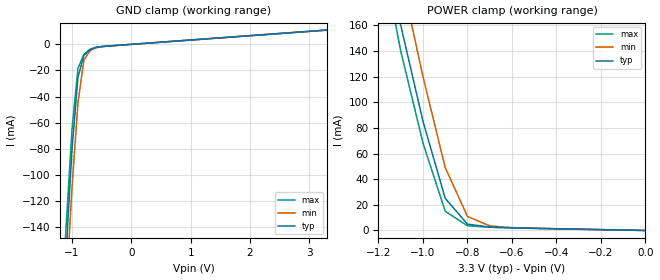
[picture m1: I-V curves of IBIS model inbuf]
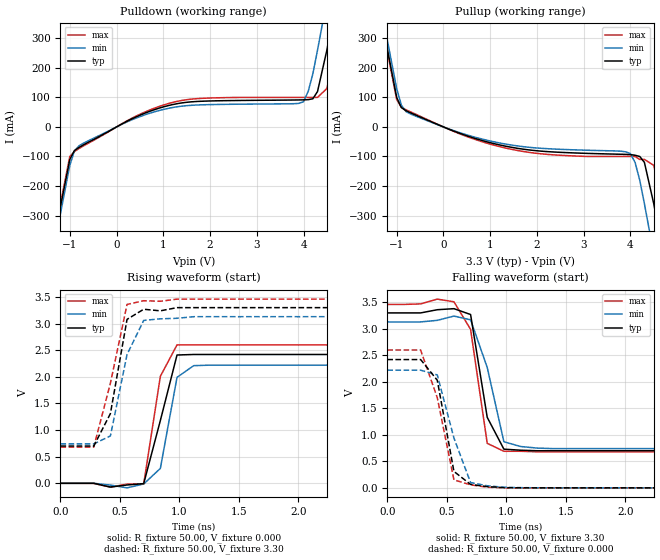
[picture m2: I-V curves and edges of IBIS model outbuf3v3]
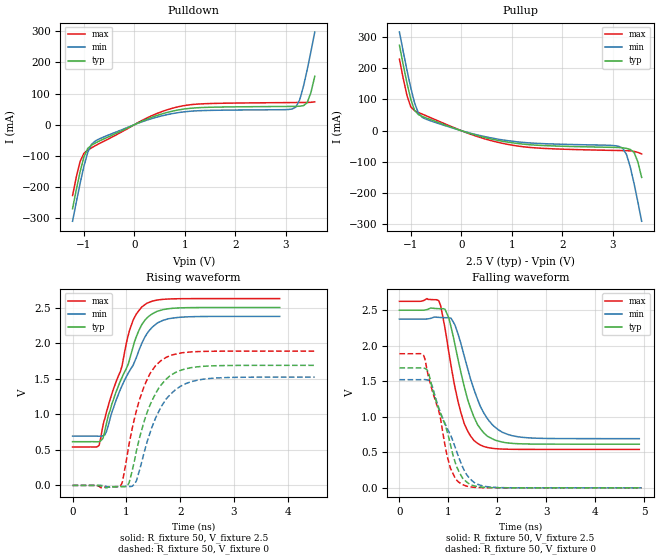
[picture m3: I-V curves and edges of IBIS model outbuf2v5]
|   Integrated Device Technology
[IBIS ver]   4.1
[File name]   5t30553.ibs
[File Rev]   1.3
|Rev history   1.3   correct temperature range information
|   1.2   add 2v5 model
|   1.1   fixed pin assignment
|   1.0   original ibis data
[Date]   June 5, 2013
[Source]   IDT
[Notes]   1. Temp typ=25C, min=85C, max=-40C 2. Ramp rates based on 50 ohm
   load
[Disclaimer] READ THESE TERMS AND CONDITIONS CAREFULLY BEFORE USING THIS
   IBIS MODEL. BY USING THIS IBIS MODEL, YOU ARE ACCEPTING AND
   AGREEING TO THESE TERMS AND CONDITIONS OF USE. Integrated
   Device Technology, Inc. ("IDT") hereby grants the user of this
   IBIS model ("User") a non-exclusive, nontransferable license
   to use this IBIS model under the following terms: The User is
   granted this license only to use the IBIS model for
   demonstration purposes only and is not granted rights to sell,
   copy (except as needed to run the IBIS model), rent, lease or
   sub-license (except for demonstration) the IBIS model in whole
   or in part, or in modified form to anyone. The User may modify
   the IBIS model to suit its specific applications, but rights
   to derivative works and such modifications shall belong to
   IDT. THIS IBIS MODEL IS PROVIDED ON AN AS IS" BASIS AND IDT
   MAKES ABSOLUTELY NO WARRANTY WITH RESPECT TO THE INFORMATION
   CONTAINED HEREIN. IDT DISCLAIMS AND USER WAIVES ALL
   WARRANTIES, EXPRESS AND IMPLIED, INCLUDING WARRANTIES OF
   MERCHAN ...
[Copyright]   Copyright 2007, Integrated Device Technology, Inc. All rights
   reserved.
|   Component 5T30553
[Component]   IDT5T30553
[Manufacturer]   Integrated Device Technology Inc.
[Package]
| variable   typ   min   max
R_pkg   40.00m   35.00m   45.00m
L_pkg   1.65nH   1.35nH   1.95nH
C_pkg   0.24pF   0.14pF   0.34pF
[Pin]  signal_name   model_name
1   VDD   POWER
2   Q0   outbuf
3   Q1   outbuf
4   GND   GND
5   ICLK   inbuf
6   Q2   outbuf
7   Q3   outbuf
8   OE   inbuf
[Model Selector]   outbuf
outbuf3v3  3.3V  LVCMOS output
outbuf2v5  2.5V  LVCMOS output
| Models and submodels in the file (3): inbuf (Input), outbuf3v3 (Output), outbuf2v5 (Output)
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|   Model inbuf
[Model]   inbuf
Model_type   Input
Vinl =   0.40V
Vinh =   2.65V
C_comp   5.50pF   5.00pF   6.00pF
[Temperature Range]   25.00   85.00   -40.00
[Voltage Range]   3.30V   3.13V   3.46V
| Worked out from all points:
|   GND clamp passes 1 mA (typ) near -0.30 V on its own axis
|   POWER clamp passes 1 mA (typ) near -0.30 V on its own axis
[GND_clamp]
| voltage   I(typ)   I(min)   I(max)
-3.3V     -2.18A     -2.2A      -2.17A
-1.2V     -240mA     -270mA     -220mA
-1.1V     -160mA     -190mA     -140mA
-1V       -80.36mA   -110mA     -64.95mA
-900mV    -25.31mA   -44.87mA   -18.41mA
-800mV    -8.54mA    -12.15mA   -7.74mA
-700mV    -4.25mA    -5.03mA    -3.87mA
-600mV    -2.38mA    -2.68mA    -2.25mA
-400mV    -1.33mA    -1.34mA    -1.33mA
3.3V      10.96mA    10.96mA    10.96mA
[POWER_clamp]
| voltage   I(typ)   I(min)   I(max)
-3.3V     2.17A      2.19A      2.16A
-1.2V     250mA      280mA      230mA
-1.1V     160mA      200mA      140mA
-1V       85.17mA    120mA      68.21mA
-900mV    25.05mA    49.08mA    14.98mA
-800mV    4.94mA     10.95mA    3.69mA
-700mV    2.68mA     3.59mA     2.48mA
-500mV    1.67mA     1.7mA      1.66mA
0V        180pA      570pA      170pA
|   Model outbuf
[Model]   outbuf3v3
Model_type   Output
Polarity   Non-Inverting
Enable   Active-High
Vmeas =   1.65V
C_comp   5.50pF   5.00pF   6.00pF
[Temperature Range]   25.00   85.00   -40.00
[Voltage Range]   3.30V   3.13V   3.46V
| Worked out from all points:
|   slope of the pulldown table from 0 to 0.495 V, typ, clamps not added: 12.6 ohm
|   slope of the pullup table from 0 to 0.495 V, typ, clamps not added: 16.7 ohm
|   rising waveform, R_fixture 50.00, V_fixture 0.000: 20-80 % time 168ps typ, 109ps min, 120ps max; typ from 0 V to 2.42 V
|   rising waveform, R_fixture 50.00, V_fixture 3.30: 20-80 % time 137ps typ, 161ps min, 172ps max; typ from 0.7 V to 3.3 V
|   falling waveform, R_fixture 50.00, V_fixture 3.30: 20-80 % time 130ps typ, 165ps min, 109ps max; typ from 3.3 V to 0.7 V
|   falling waveform, R_fixture 50.00, V_fixture 0.000: 20-80 % time 118ps typ, 181ps min, 166ps max; typ from 2.42 V to 0 V
[Pulldown]
| voltage   I(typ)   I(min)   I(max)
-3.3V     -2.18A     -2.2A      -2.17A
-1.5V     -510mA     -540mA     -500mA
-1V       -110mA     -130mA     -100mA
-800mV    -69.02mA   -63.67mA   -72.8mA
800mV     57.94mA    50.69mA    62.96mA
4V        91.72mA    85.55mA    100mA
4.1V      92.42mA    120mA      100mA
4.3V      120mA      260mA      100mA
4.5V      260mA      430mA      130mA
4.7V      430mA      610mA      270mA
4.9V      610mA      790mA      450mA
6.6V      2.18A      2.35A      2.01A
[Pullup]
| voltage   I(typ)   I(min)   I(max)
-3.3V     2.17A      2.19A      2.16A
-1.5V     510mA      540mA      500mA
-900mV    65.55mA    73.95mA    66.71mA
0V        180pA      560pA      160pA
1.7V      -75.17mA   -66.67mA   -82.91mA
4V        -93.72mA   -90.2mA    -100mA
4.1V      -95.8mA    -120mA     -100mA
4.3V      -120mA     -260mA     -110mA
4.5V      -260mA     -430mA     -130mA
4.7V      -430mA     -600mA     -270mA
4.9V      -610mA     -780mA     -440mA
6.6V      -2.19A     -2.36A     -2.02A
[Ramp]
| variable   typ   min   max
dV/dt_r   1.45/87.35p   1.33/88.23p   1.56/77.67p
dV/dt_f   1.56/97.64p   1.44/0.12n   1.67/89.32p
R_load = 50.00
[Rising Waveform]
R_fixture = 50.00
V_fixture = 0.000
V_fixture_min = 0.000
V_fixture_max = 0.000
| time   V(typ)   V(min)   V(max)
0s        0V         0V         0V
280ps     380uV      270uV      -1.89mV
420ps     -70.83mV   -33.33mV   -72.2mV
560ps     -31.68mV   -85.61mV   -14.5mV
700ps     -5.79mV    -12.69mV   -12.02mV
840ps     1.18V      280mV      2.01V
980ps     2.41V      1.99V      2.6V
1.12ns    2.42V      2.21V      2.6V
1.26ns    2.42V      2.22V      2.6V
7ns       2.42V      2.22V      2.6V
[Rising Waveform]
R_fixture = 50.00
V_fixture = 3.30
V_fixture_min = 3.13
V_fixture_max = 3.46
| time   V(typ)   V(min)   V(max)
0s        700mV      740mV      680mV
280ps     700mV      740mV      680mV
420ps     1.31V      890mV      1.88V
560ps     3.08V      2.42V      3.36V
700ps     3.27V      3.06V      3.43V
840ps     3.24V      3.09V      3.42V
980ps     3.3V       3.1V       3.46V
1.12ns    3.3V       3.13V      3.46V
7ns       3.3V       3.13V      3.46V
[Falling Waveform]
R_fixture = 50.00
V_fixture = 3.30
V_fixture_min = 3.13
V_fixture_max = 3.46
| time   V(typ)   V(min)   V(max)
0s        3.3V       3.13V      3.46V
280ps     3.3V       3.13V      3.47V
420ps     3.36V      3.16V      3.56V
560ps     3.38V      3.24V      3.51V
700ps     3.27V      3.17V      2.99V
840ps     1.33V      2.27V      840mV
980ps     730mV      870mV      690mV
1.12ns    710mV      780mV      690mV
1.4ns     700mV      740mV      680mV
7ns       700mV      740mV      680mV
[Falling Waveform]
R_fixture = 50.00
V_fixture = 0.000
V_fixture_min = 0.000
V_fixture_max = 0.000
| time   V(typ)   V(min)   V(max)
0s        2.42V      2.22V      2.6V
280ps     2.42V      2.22V      2.6V
420ps     2.03V      2.13V      1.7V
560ps     310mV      940mV      150mV
700ps     64.38mV    100mV      57.17mV
840ps     23.39mV    39.34mV    11.78mV
980ps     4.1mV      11.18mV    1.54mV
1.26ns    320uV      820uV      49.82uV
7ns       2.26uV     -670nV     1.97uV
[Model]   outbuf2v5
Model_type   Output
Polarity   Non-Inverting
|   typ   min   max
C_comp   2pF   1.5pF   2.5pF
Vmeas = 2.00V
Rref = 50
Cref = 0
Vref = 1.25V
|   typ   min   max
[Voltage range]   2.5V   2.375V   2.625V
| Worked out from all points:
|   slope of the pulldown table from 0 to 0.375 V, typ, clamps not added: 14.7 ohm
|   slope of the pullup table from 0 to 0.375 V, typ, clamps not added: 20.7 ohm
|   rising waveform, R_fixture 50, V_fixture 2.5: 20-80 % time 535ps typ, 582ps min, 466ps max; typ from 0.615 V to 2.5 V
|   falling waveform, R_fixture 50, V_fixture 2.5: 20-80 % time 423ps typ, 493ps min, 360ps max; typ from 2.5 V to 0.615 V
|   rising waveform, R_fixture 50, V_fixture 0: 20-80 % time 440ps typ, 466ps min, 395ps max; typ from 0 V to 1.69 V
|   falling waveform, R_fixture 50, V_fixture 0: 20-80 % time 458ps typ, 525ps min, 387ps max; typ from 1.69 V to 0 V
[Pulldown]
|Voltage   I (typ)   I (min)   I (max)
|Note, modeling breaks down at 250mA and above.  This is well beyond the functional   |
|operating range of the device.  Should this scenario occur, catastrophic failure and   |
|possible damage to the device and/or board is of higher concern than the I-V curve   |
|behavior.  The IBIS checker will flag currents in excess of 10A with warnings.  Lines   |
|with currents in excess of 0.35 A have been commented out.  The points still remain|
|available to the user if the user desires to use them.   |
|-2.50000e+00   -1.43294e+00   -1.46452e+00   -1.40036e+00
|-2.42500e+00   -1.36296e+00   -1.39507e+00   -1.32977e+00
|-2.35000e+00   -1.29305e+00   -1.32571e+00   -1.25925e+00
|-2.27500e+00   -1.22322e+00   -1.25643e+00   -1.18880e+00
|-2.20000e+00   -1.15348e+00   -1.18724e+00   -1.11843e+00
|-2.12500e+00   -1.08384e+00   -1.11817e+00   -1.04815e+00
|-2.05000e+00   -1.01432e+00   -1.04922e+00   -9.77977e-01
|-1.97500e+00   -9.44937e-01   -9.80409e-01   -9.07925e-01
|-1.90000e+00   -8.75705e-01   -9.11761e-01   -8.38016e-01
|-1.82500e+00   -8.06655e-01   -8.43301e-01   -7.68277e-01
|-1.75000e+00   -7.37821e-01   -7.75060e-01   -6.98745e-01
|-1.67500e+00   -6.69249e-01   -7.07081e-01   -6.29468e-01
|-1.60000e+00   -6.00999e-01   -6.39417e-01   -5.60513e-01
|-1.52500e+00   -5.33155e-01   -5.72143e-01   -4.91977e-01
|-1.45000e+00   -4.65837e-01   -5.05359e-01   -4.24009e-01
|-1.37500e+00   -3.99226e-01   -4.39208e-01   -3.56847e-01
|-1.30000e+00   -3.33611e-01   -3.73906e-01   -2.90914e-01
-1.225V   -269.5mA   -309.8mA   -227.1mA
-1.075V   -150.7mA   -188mA     -117.6mA
-1V       -103.5mA   -133.6mA   -91.79mA
-925mV    -76.41mA   -89.37mA   -82mA
-775mV    -58.87mA   -52.28mA   -67.28mA
275mV     19.49mA    16.07mA    23.65mA
875mV     47.36mA    38.83mA    57.69mA
3.125V    58.64mA    50.22mA    70.97mA
3.275V    59.3mA     79.43mA    71.16mA
3.425V    70.52mA    176.3mA    71.44mA
3.5V      103.9mA    235.3mA    71.81mA
3.575V    155.2mA    297.2mA    73.4mA
| 3.65000e+00   2.14000e-01   3.60803e-01   8.80326e-02
| 3.72500e+00   2.76351e-01   4.25612e-01   1.32256e-01
| 3.80000e+00   3.40691e-01   4.91258e-01   1.90161e-01
| 3.87500e+00   4.06282e-01   5.57528e-01   2.53007e-01
| 3.95000e+00   4.72725e-01   6.24279e-01   3.18194e-01
| 4.02500e+00   5.39786e-01   6.91413e-01   3.84717e-01
| 4.10000e+00   6.07310e-01   7.58858e-01   4.52098e-01
| 4.17500e+00   6.75198e-01   8.26560e-01   5.20072e-01
| 4.25000e+00   7.43376e-01   8.94477e-01   5.88481e-01
| 4.32500e+00   8.11792e-01   9.62579e-01   6.57220e-01
| 4.40000e+00   8.80406e-01   1.03084e+00   7.26220e-01
| 4.47500e+00   9.49187e-01   1.09924e+00   7.95430e-01
| 4.55000e+00   1.01811e+00   1.16776e+00   8.64812e-01
| 4.62500e+00   1.08716e+00   1.23638e+00   9.34340e-01
| 4.70000e+00   1.15632e+00   1.30511e+00   1.00399e+00
| 4.77500e+00   1.22557e+00   1.37392e+00   1.07375e+00
| 4.85000e+00   1.29490e+00   1.44280e+00   1.14359e+00
| 4.92500e+00   1.36432e+00   1.51176e+00   1.21352e+00
| 5.00000e+00   1.43380e+00   1.58078e+00   1.28352e+00
[Pullup]
|Voltage   I (typ)   I (min)   I (max)
|Note, modeling breaks down at 250mA and above.  This is well beyond the functional   |
|operating range of the device.  Should this scenario occur, catastrophic failure and   |
|possible damage to the device and/or board is of higher concern than the I-V curve   |
|behavior.  The IBIS checker will flag currents in excess of 10A with warnings.  Lines   |
|with currents in excess of 0.35 A have been commented out.  The points still remain|
|available to the user if the user desires to use them.   |
|-2.50000e+00   1.43050e+00   1.46286e+00   1.39670e+00
|-2.42500e+00   1.36103e+00   1.39396e+00   1.32660e+00
|-2.35000e+00   1.29162e+00   1.32512e+00   1.25657e+00
|-2.27500e+00   1.22228e+00   1.25638e+00   1.18660e+00
|-2.20000e+00   1.15304e+00   1.18772e+00   1.11671e+00
|-2.12500e+00   1.08389e+00   1.11917e+00   1.04690e+00
|-2.05000e+00   1.01484e+00   1.05073e+00   9.77186e-01
|-1.97500e+00   9.45925e-01   9.82431e-01   9.07587e-01
|-1.90000e+00   8.77150e-01   9.14280e-01   8.38120e-01
|-1.82500e+00   8.08545e-01   8.46305e-01   7.68808e-01
|-1.75000e+00   7.40137e-01   7.78536e-01   6.99683e-01
|-1.67500e+00   6.71968e-01   7.11009e-01   6.30786e-01
|-1.60000e+00   6.04091e-01   6.43774e-01   5.62175e-01
|-1.52500e+00   5.36579e-01   5.76896e-01   4.93932e-01
|-1.45000e+00   4.69532e-01   5.10464e-01   4.26177e-01
|-1.37500e+00   4.03103e-01   4.44604e-01   3.59099e-01
|-1.30000e+00   3.37526e-01   3.79499e-01   2.93022e-01
-1.225V   273.2mA    315.4mA    228.6mA
-1.075V   152mA      192.7mA    112.2mA
-1V       100.3mA    136.7mA    75.7mA
-925mV    65.04mA    88.66mA    64.18mA
-850mV    51.53mA    56.45mA    58.43mA
-775mV    45.69mA    42.91mA    53.13mA
200mV     -10.21mA   -8.901mA   -12.27mA
950mV     -37.44mA   -32.67mA   -44.8mA
3.125V    -53.99mA   -50.49mA   -63.58mA
3.275V    -56.8mA    -76.28mA   -64.09mA
3.425V    -69.68mA   -169.4mA   -66.35mA
3.575V    -149.5mA   -290mA     -74.53mA
| 3.65000e+00   -2.07857e-01   -3.53795e-01   -8.82396e-02
| 3.72500e+00   -2.70185e-01   -4.18918e-01   -1.28976e-01
| 3.80000e+00   -3.34712e-01   -4.84944e-01   -1.85784e-01
| 3.87500e+00   -4.00602e-01   -5.51637e-01   -2.48418e-01
| 3.95000e+00   -4.67410e-01   -6.18840e-01   -3.13718e-01
| 4.02500e+00   -5.34877e-01   -6.86449e-01   -3.80505e-01
| 4.10000e+00   -6.02837e-01   -7.54385e-01   -4.48228e-01
| 4.17500e+00   -6.71179e-01   -8.22591e-01   -5.16592e-01
| 4.25000e+00   -7.39828e-01   -8.91022e-01   -5.85422e-01
| 4.32500e+00   -8.08725e-01   -9.59645e-01   -6.54603e-01
| 4.40000e+00   -8.77828e-01   -1.02843e+00   -7.24060e-01
| 4.47500e+00   -9.47105e-01   -1.09737e+00   -7.93737e-01
| 4.55000e+00   -1.01653e+00   -1.16642e+00   -8.63597e-01
| 4.62500e+00   -1.08609e+00   -1.23559e+00   -9.33607e-01
| 4.70000e+00   -1.15575e+00   -1.30486e+00   -1.00375e+00
| 4.77500e+00   -1.22552e+00   -1.37422e+00   -1.07399e+00
| 4.85000e+00   -1.29537e+00   -1.44365e+00   -1.14434e+00
| 4.92500e+00   -1.36530e+00   -1.51316e+00   -1.21476e+00
| 5.00000e+00   -1.43530e+00   -1.58273e+00   -1.28526e+00
[Ramp]
|   typ   min   max
dV/dt_r   1.131/0.534n   1.01/0.582n   1.25/0.466n
dV/dt_f   1.15/0.428n  1.027/0.497n   1.273/0.364n
R_load =   50.0000
[Rising Waveform]
R_fixture = 50
V_fixture = 2.5   |Vcc_typ
V_fixture_min = 2.375 |Vcc_min
V_fixture_max = 2.625 |Vcc_max
C_fixture = 0.0p
| Time   typ   min   max
0s        614.6mV    692.4mV    540.5mV
493.4ps   613.9mV    691.4mV    562.7mV
566.2ps   662.7mV    698.8mV    845.9mV
614.5ps   818.8mV    732.3mV    984.9mV
918.8ps   1.517V     1.4V       1.677V
1.057ns   1.765V     1.606V     2.174V
1.186ns   2.092V     1.798V     2.41V
1.383ns   2.354V     2.132V     2.56V
1.871ns   2.49V      2.352V     2.622V
3.85ns    2.5V       2.375V     2.625V
[Falling Waveform]
R_fixture = 50
V_fixture = 2.5   |Vcc_typ
V_fixture_min = 2.375 |Vcc_min
V_fixture_max = 2.625 |Vcc_max
C_fixture = 0.0p
| Time   typ   min   max
0s        2.5V       2.375V     2.625V
804.5ps   2.522V     2.4V       2.631V
1.008ns   2.394V     2.395V     1.913V
1.133ns   2.022V     2.294V     1.419V
1.251ns   1.638V     2.042V     1.069V
1.397ns   1.236V     1.671V     795.5mV
1.597ns   888.8mV    1.244V     626.4mV
1.901ns   689mV      886mV      555.9mV
2.301ns   626.1mV    734.2mV    542.3mV
4.901ns   614.6mV    692.4mV    540.5mV
[Rising Waveform]
R_fixture = 50
V_fixture = 0
C_fixture = 0.0p
| Time   typ   min   max
0s        82.06pV    15.73nV    12.89pV
889.1ps   -16.05mV   -16.86mV   -9.346mV
927.5ps   -16.07mV   -15.8mV    51.81mV
1.052ns   39.3mV     -14.34mV   585mV
1.188ns   485.5mV    67.69mV    1.052V
1.332ns   905.1mV    468.1mV    1.397V
1.543ns   1.291V     946.9mV    1.683V
1.743ns   1.495V     1.218V     1.801V
2.402ns   1.672V     1.49V      1.882V
4.502ns   1.687V     1.522V     1.887V
[Falling Waveform]
R_fixture = 50
V_fixture = 0
C_fixture = 0.0p
| Time   typ   min   max
0s        1.687V     1.522V     1.887V
491.1ps   1.688V     1.523V     1.867V
569.5ps   1.655V     1.518V     1.638V
641.8ps   1.482V     1.48V      1.44V
802.2ps   1.114V     1.13V      1.087V
1.043ns   606.5mV    748.1mV    275.7mV
1.291ns   134.8mV    292.7mV    45.4mV
1.491ns   34.43mV    95.6mV     9.42mV
1.749ns   7.371mV    19.56mV    1.268mV
4.948ns   5.711nV    -56.82nV   -167.8nV
